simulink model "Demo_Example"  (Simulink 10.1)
settings: Solver=FixedStepDiscrete  StartTime=0.0  StopTime=100  FixedStep=1  RelTol=1e-3

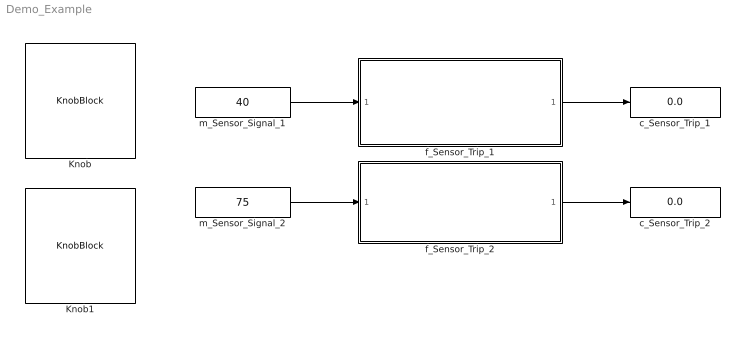
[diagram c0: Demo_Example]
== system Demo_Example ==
  Knob : KnobBlock
  Knob1 : KnobBlock
  c_Sensor_Trip_1 : Display
  c_Sensor_Trip_2 : Display
  f_Sensor_Trip_1 : Subsystem
  f_Sensor_Trip_2 : Subsystem
  m_Sensor_Signal_1 : Constant  Value=40  OutDataTypeStr=int16
  m_Sensor_Signal_2 : Constant  Value=75  OutDataTypeStr=int16
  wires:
  m_Sensor_Signal_2/1 -> f_Sensor_Trip_2/1(m_Sensor_Signal_2)
  m_Sensor_Signal_1/1 -> f_Sensor_Trip_1/1(m_Sensor_Signal_1)
  f_Sensor_Trip_2/1(c_Sensor_Trip_2) -> c_Sensor_Trip_2/1
  f_Sensor_Trip_1/1(c_Sensor_Trip_1) -> c_Sensor_Trip_1/1

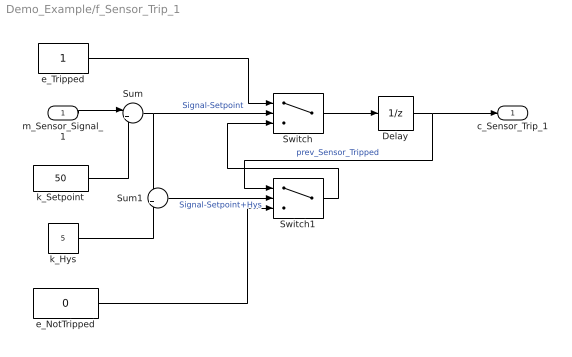
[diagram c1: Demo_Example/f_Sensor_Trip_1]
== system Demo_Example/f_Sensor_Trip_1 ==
  m_Sensor_Signal_1 : Inport  OutDataTypeStr=int16
  Delay : UnitDelay  SampleTime=-1  HasFrameUpgradeWarning=on
  Sum : Sum  Inputs=|+-
  Sum1 : Sum
  Switch : Switch  OutDataTypeStr=boolean
  Switch1 : Switch  OutDataTypeStr=boolean
  e_NotTripped : Constant  Value=0  OutDataTypeStr=boolean
  e_Tripped : Constant  OutDataTypeStr=boolean
  k_Hys : Constant  Value=5  OutDataTypeStr=int16
  k_Setpoint : Constant  Value=50  OutDataTypeStr=int16
  c_Sensor_Trip_1 : Outport  OutDataTypeStr=boolean
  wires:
  m_Sensor_Signal_1/1 -> Sum/1
  Sum/1 -> Switch/2, Sum1/1  "Signal-Setpoint"
  e_Tripped/1 -> Switch/1
  Switch/1 -> Delay/1
  Delay/1 -> Switch1/1, c_Sensor_Trip_1/1  "prev_Sensor_Tripped"
  Switch1/1 -> Switch/3
  k_Hys/1 -> Sum1/2
  Sum1/1 -> Switch1/2  "Signal-Setpoint+Hys"
  e_NotTripped/1 -> Switch1/3
  k_Setpoint/1 -> Sum/2

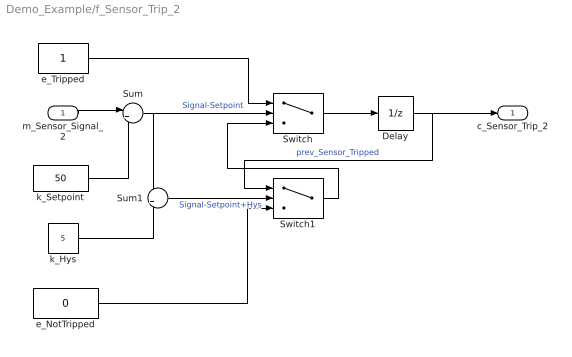
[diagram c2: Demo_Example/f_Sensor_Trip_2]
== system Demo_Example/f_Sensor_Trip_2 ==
  m_Sensor_Signal_2 : Inport  OutDataTypeStr=int16
  Delay : UnitDelay  SampleTime=-1  HasFrameUpgradeWarning=on
  Sum : Sum  Inputs=|+-
  Sum1 : Sum
  Switch : Switch  OutDataTypeStr=boolean
  Switch1 : Switch  OutDataTypeStr=boolean
  e_NotTripped : Constant  Value=0  OutDataTypeStr=boolean
  e_Tripped : Constant  OutDataTypeStr=boolean
  k_Hys : Constant  Value=5  OutDataTypeStr=int16
  k_Setpoint : Constant  Value=50  OutDataTypeStr=int16
  c_Sensor_Trip_2 : Outport  OutDataTypeStr=boolean
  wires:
  k_Setpoint/1 -> Sum/2
  e_NotTripped/1 -> Switch1/3
  Sum1/1 -> Switch1/2  "Signal-Setpoint+Hys"
  k_Hys/1 -> Sum1/2
  Switch1/1 -> Switch/3
  Delay/1 -> c_Sensor_Trip_2/1, Switch1/1  "prev_Sensor_Tripped"
  Switch/1 -> Delay/1
  e_Tripped/1 -> Switch/1
  Sum/1 -> Sum1/1, Switch/2  "Signal-Setpoint"
  m_Sensor_Signal_2/1 -> Sum/1
